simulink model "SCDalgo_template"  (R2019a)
settings: configuration reference "configurationSettings" (kept in a data dictionary, not in this file)
undefined symbols (not defined in the file or in its folder): ProductionState, QualityTag, SCDalgo_template_fp, SCDalgo_template_tp, SCDsignal_example_1, SCDsignal_example_3, Value

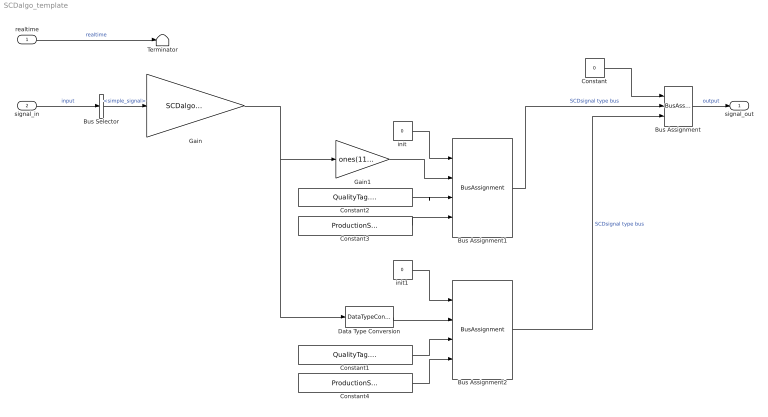
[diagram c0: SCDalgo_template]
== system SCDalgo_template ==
  realtime : Inport  OutDataTypeStr=single  PortDimensions=1  SampleTime=SCDalgo_template_fp.timing.dt  Interpolate=off
  signal_in : Inport  Port=2  OutDataTypeStr=Bus: SCDalgo_template_inBus  PortDimensions=1  SampleTime=SCDalgo_template_fp.timing.dt  Interpolate=off
  Bus Assignment : BusAssignment  AssignedSignals=SCDsignal_example_1,SCDsignal_example_3
  Bus Assignment1 : BusAssignment  AssignedSignals=Value,QualityTag,ProductionState
  Bus Assignment2 : BusAssignment  AssignedSignals=Value,QualityTag,ProductionState
  Bus Selector : BusSelector  OutputSignals=simple_signal
  Constant : Constant  Value=0  OutDataTypeStr=Bus: SCDalgo_template_outBus
  Constant1 : Constant  Value=QualityTag.INVALID  OutDataTypeStr=Enum: QualityTag
  Constant2 : Constant  Value=QualityTag.GOOD  OutDataTypeStr=Enum: QualityTag
  Constant3 : Constant  Value=ProductionState.RUNNING  OutDataTypeStr=Enum: ProductionState
  Constant4 : Constant  Value=ProductionState.OUTDATED  OutDataTypeStr=Enum: ProductionState
  Data Type Conversion : DataTypeConversion  OutDataTypeStr=int32
  Gain : Gain  Gain=SCDalgo_template_tp.gain
  Gain1 : Gain  Gain=ones(11,1)
  Terminator : Terminator
  init : Constant  Value=0  OutDataTypeStr=Bus: SCDBus_single_11_Vector
  init1 : Constant  Value=0  OutDataTypeStr=Bus: SCDBus_int32_Scalar
  signal_out : Outport  OutDataTypeStr=Bus: SCDalgo_template_outBus
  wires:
  signal_in/1 -> Bus Selector/1  "input"
  Bus Selector/1 -> Gain/1  "<simple_signal>"
  Constant/1 -> Bus Assignment/1
  realtime/1 -> Terminator/1  "realtime"
  Bus Assignment/1 -> signal_out/1  "output"
  init/1 -> Bus Assignment1/1
  Bus Assignment1/1 -> Bus Assignment/2  "SCDsignal type bus"
  Constant2/1 -> Bus Assignment1/3
  Constant3/1 -> Bus Assignment1/4
  Gain/1 -> Gain1/1, Data Type Conversion/1
  Gain1/1 -> Bus Assignment1/2
  init1/1 -> Bus Assignment2/1
  Data Type Conversion/1 -> Bus Assignment2/2
  Constant1/1 -> Bus Assignment2/3
  Constant4/1 -> Bus Assignment2/4
  Bus Assignment2/1 -> Bus Assignment/3  "SCDsignal type bus"
